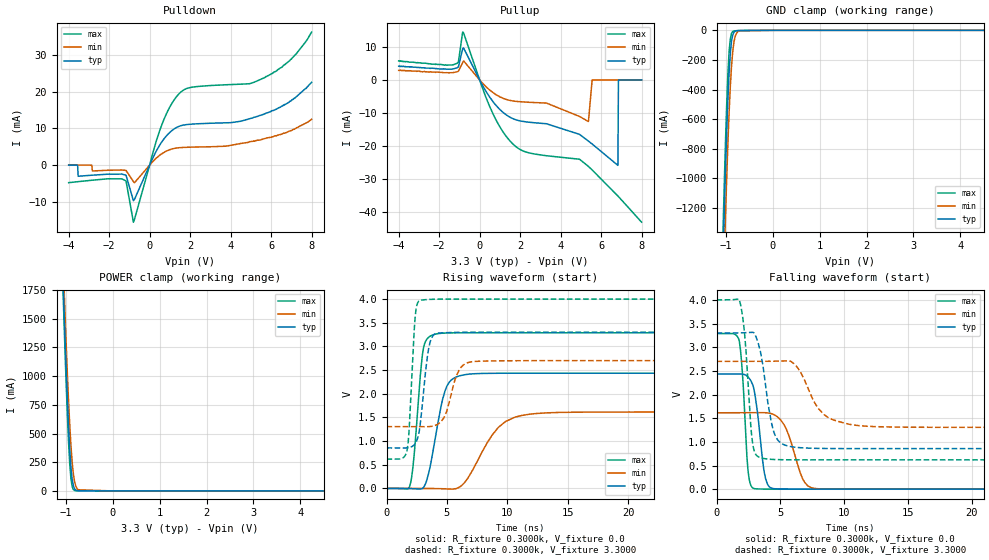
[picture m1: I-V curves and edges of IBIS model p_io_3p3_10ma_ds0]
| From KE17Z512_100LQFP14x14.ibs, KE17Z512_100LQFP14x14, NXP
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[Model] p_io_3p3_10ma_ds0
|   Model p_io_3p3_10ma_ds0
| This model was characterised for following simulation conditions:
| External (pad) voltage:
|   - Typ: 3.3V,   - Min: 2.7V,   - Max: 4.0V
| Library cells for typ/min/max conditions are connected as defined below:
|  pad - External Pad
|  ipp_do_lv - Core Input
|  ipp_obe_lv - Output Buffer Enable
|  abt_close_nor_rst_mv - vdde
|  dvdd - dvdd
|  dvss - dvss
|  esd_boost - vdde
|  ipp_dse_lv - dvss
|  ipp_ina_280_mv - NC
|  ipp_ina_40_a_mv - NC
|  ipp_ina_40_b_mv - NC
|  ipp_ina_40_c_mv - NC
|  ipp_ina_40_d_mv - NC
|  ipp_ina_40_e_mv - NC
|  ipp_ina_40_f_mv - NC
|  ipp_ina_40_g_mv - NC
|  ipp_ina_40_h_mv - NC
|  ipp_ind_lv - NC
|  ipp_sre_lv - dvss
|  vdde - vdde
|  vsse - vsse
| All other pins connected to ground
Model_type I/O
Polarity   Non-Inverting
Enable   Active-High
Vinl =   0.9900V
Vinh =   2.3100V
Vmeas =  1.6500V
Cref =   50.0000F
C_comp   1.9352pF   1.8468pF   2.0590pF
[Model Spec]
| variable   typ   min   max
Vinh   2.3100V   1.8900V   2.8000V
Vinl   0.9900V   0.8100V   1.2000V
S_overshoot_high   3.6000V   3.0000V   4.3000V
S_overshoot_low   -0.3000V   -0.3000V   -0.3000V
Vmeas   1.6500V   1.3500V   2.0000V
[Temperature Range]   25.0000   0.1250k   -40.0000
[Voltage Range]   3.3000V   2.7000V   4.0000V
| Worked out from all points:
|   slope of the pulldown table from 0 to 0.495 V, typ, clamps not added: 90.9 ohm
|   slope of the pullup table from 0 to 0.495 V, typ, clamps not added: 95.3 ohm
|   rising waveform, R_fixture 0.3000k, V_fixture 0.0: 20-80 % time 1.08ns typ, 2.28ns min, 618ps max; typ from 0 V to 2.43 V
|   rising waveform, R_fixture 0.3000k, V_fixture 3.3000: 20-80 % time 615ps typ, 950ps min, 407ps max; typ from 0.857 V to 3.3 V
|   falling waveform, R_fixture 0.3000k, V_fixture 0.0: 20-80 % time 627ps typ, 1.16ns min, 408ps max; typ from 2.43 V to 0 V
|   falling waveform, R_fixture 0.3000k, V_fixture 3.3000: 20-80 % time 848ps typ, 1.71ns min, 512ps max; typ from 3.3 V to 0.857 V
[Pulldown]
|Voltage   I(typ)   I(min)   I(max)
-4V       0A         10uA       -4.79mA
-3.558V   -10uA      10uA       -4.53mA
-3.532V   -3.04mA    10uA       -4.51mA
-1.166V   -2.774mA   -1.45mA    -4.321mA
-802mV    -9.71mA    -4.496mA   -15.58mA
498mV     5.474mA    2.695mA    9.451mA
1.434V    10.54mA    4.733mA    19.35mA
2.006V    11.15mA    4.894mA    21.17mA
4.944V    12.67mA    6.4mA      22.22mA
5.724V    14.1mA     7.3mA      24mA
6.998V    17.6mA     9.4mA      28.9mA
8V        22.6mA     12.5mA     36.3mA
[Pullup]
|Voltage   I(typ)   I(min)   I(max)
-4V       4.2mA      2.9mA      5.8mA
-1.1V     3.73mA     2.5mA      5.09mA
-814mV    9.683mA    5.577mA    14.47mA
486mV     -5.117mA   -3.013mA   -7.937mA
1.526V    -11.4mA    -6.246mA   -18.7mA
3.3V      -13.29mA   -7.013mA   -23.01mA
4.932V    -16.52mA   -11.08mA   -24.07mA
5.374V    -18.57mA   -12.63mA   -26.26mA
5.556V    -19.44mA   0A         -27.32mA
6.83V     -25.93mA   10uA       -35.25mA
6.856V    -20uA      10uA       -35.42mA
8V        10uA       10uA       -43.19mA
[GND_clamp]
|Voltage   I(typ)   I(min)   I(max)
-4V       -44.22A    -44.15A    -44.31A
-1.062V   -1.538A    -1.84A     -1.36A
-1.036V   -1.238A    -1.547A    -1.053A
-1.01V    -956.2mA   -1.268A    -766.3mA
-958mV    -472.3mA   -768mA     -297.7mA
-932mV    -288.7mA   -557.4mA   -144.7mA
-906mV    -155.5mA   -380.4mA   -57.41mA
-880mV    -73.51mA   -241.5mA   -20.32mA
-828mV    -13.22mA   -77.7mA    -4.19mA
-776mV    -3.062mA   -20.44mA   -2.572mA
-698mV    -1.117mA   -2.814mA   -1.68mA
8V        0A         0A         0A
[POWER_clamp]
|Voltage   I(typ)   I(min)   I(max)
-4V       44.89A     44.69A     45.07A
-1.074V   1.999A     2.184A     1.905A
-1.048V   1.679A     1.877A     1.575A
-1.022V   1.371A     1.58A      1.256A
-970mV    807.7mA    1.033A     674.4mA
-918mV    359.9mA    574.8mA    234.3mA
-892mV    203mA      392.8mA    103.5mA
-866mV    99.48mA    249.2mA    36.93mA
-814mV    17.16mA    79.21mA    3.9mA
-736mV    1.301mA    9.822mA    753.1uA
0V        71.73pA    1.381nA    67.44pA
8V        0A         0A         0A
[Ramp]
| variable   typ   min   max
dV/dt_r  1.4602/1.0838n   0.9683/2.2799n   1.9729/0.6182n
dV/dt_f  1.4660/0.8478n   0.8362/1.7102n   2.0284/0.5117n
R_load = 0.3000k
[Rising Waveform]
R_fixture= 0.3000k
V_fixture= 0.0
V_fixture_min= 0.0
V_fixture_max= 0.0
|time   V(typ)   V(min)   V(max)
0s        106.2pV    30.82nV    370.3pV
1.909ns   -2.548mV   95.37uV    37.55mV
2.282ns   -5.975mV   129.3uV    694.4mV
2.976ns   278.7uV    -25.48uV   2.834V
3.937ns   915.6mV    -2.42mV    3.253V
4.997ns   2.162V     -10.87mV   3.284V
6.36ns    2.398V     98.12mV    3.288V
9.264ns   2.433V     1.29V      3.288V
11.18ns   2.433V     1.54V      3.288V
40ns      2.434V     1.614V     3.288V
[Rising Waveform]
R_fixture= 0.3000k
V_fixture= 3.3000
V_fixture_min= 2.7000
V_fixture_max= 4.0000
|time   V(typ)   V(min)   V(max)
0s        856.6mV    1.306V     619.2mV
1.701ns   855.8mV    1.306V     804.6mV
1.845ns   860.9mV    1.306V     1.138V
2.381ns   951.8mV    1.304V     3.651V
2.747ns   1.277V     1.303V     3.968V
3.475ns   2.937V     1.304V     3.992V
4.151ns   3.274V     1.344V     3.998V
5.997ns   3.297V     2.494V     4V
7.08ns    3.299V     2.677V     4V
40ns      3.3V       2.7V       4V
[Falling Waveform]
R_fixture= 0.3000k
V_fixture= 0.0
V_fixture_min= 0.0
V_fixture_max= 0.0
|time   V(typ)   V(min)   V(max)
0s        2.434V     1.614V     3.288V
1.753ns   2.435V     1.614V     3.162V
2.02ns    2.432V     1.614V     2.481V
2.489ns   2.365V     1.613V     339.9mV
2.969ns   2.058V     1.614V     10.45mV
3.738ns   356.5mV    1.616V     1.96mV
4.358ns   16.63mV    1.59V      786.2uV
6.904ns   417.9uV    142.8mV    43.92uV
7.622ns   203.8uV    17.7mV     25.27uV
40ns      2.749uV    5.689uV    1.304uV
[Falling Waveform]
R_fixture= 0.3000k
V_fixture= 3.3000
V_fixture_min= 2.7000
V_fixture_max= 4.0000
|time   V(typ)   V(min)   V(max)
0s        3.3V       2.7V       4V
1.8ns     3.3V       2.7V       3.986V
2.189ns   3.304V     2.7V       3.316V
2.792ns   3.313V     2.7V       1.037V
3.465ns   2.866V     2.7V       662.3mV
4.501ns   1.197V     2.704V     626.7mV
5.681ns   906.7mV    2.708V     620.5mV
8.425ns   859.6mV    1.574V     619.3mV
10.78ns   857.1mV    1.354V     619.3mV
40ns      856.6mV    1.306V     619.3mV
